FUNCTION_BLOCK FB_Count IMPLEMENTS I_Count
VAR
	i,k: INT;
	max_i:INT:=755;
	max_k: INT:=2265;
END_VAR

{warning 'add method implementation'}
METHOD M_Count : INT
VAR_INPUT
	bEnable	: BOOL;
END_VAR
VAR_OUTPUT
	i_Wert	: INT;
	k_Wert	: INT;
END_VAR
IF bEnable THEN
	i:=i+1;
	IF i>=max_i THEN
		i:=0;
	END_IF
	k:=k+1;
	IF k>=max_k THEN
		k:=0;
	END_IF
	i_Wert:=i;
	k_Wert:=k;
END_IF
END_METHOD

{warning 'add property implementation'}
PROPERTY P_Max_i : INT
GET
P_Max_i:=max_i;
END_GET
SET
max_i:=P_Max_i;
END_SET
END_PROPERTY

{warning 'add property implementation'}
PROPERTY P_Max_k : INT
GET
P_Max_k:=max_k;
END_GET
SET
max_k:=P_Max_k;
END_SET
END_PROPERTY

END_FUNCTION_BLOCK
